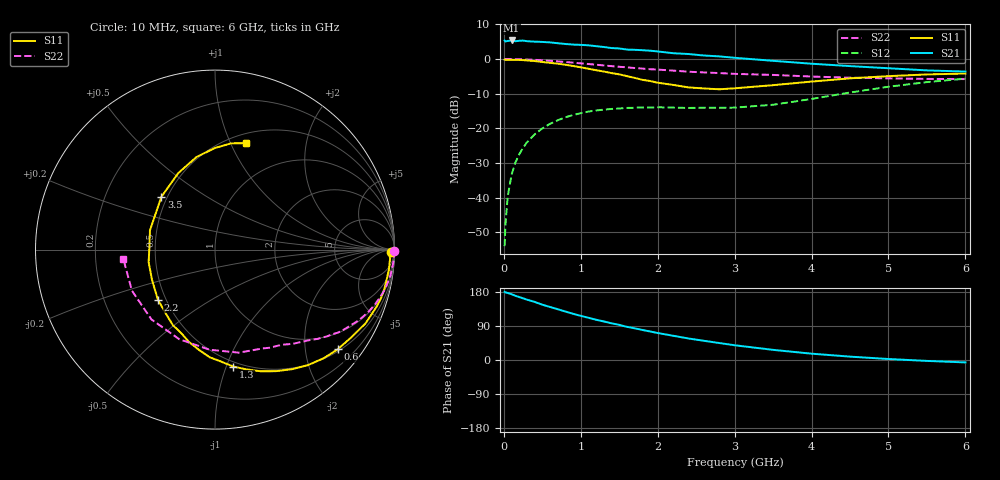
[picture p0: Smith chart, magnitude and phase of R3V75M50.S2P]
! SIEMENS Small Signal Semiconductors
! BFR181
! Si NPN RF Bipolar Junction Transistor in SOT23
! VCE = 0.75 V  IC = 0.5 mA
! Common Emitter S-Parameters:  May  1996
# GHz  S  MA  R  50
!  f  S11  S21  S12  S22
! GHz  MAG  ANG  MAG  ANG  MAG  ANG  MAG  ANG
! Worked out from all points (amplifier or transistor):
!   36 points, 10 MHz to 6 GHz, reference 50 ohm
!   highest |S21| = 5.3 dB at 100 MHz (marker M1)
!   |S21| within 3 dB of that: start of sweep to 1.923 GHz
!   unconditionally stable (mu >= 1): 2.261 GHz to 4.407 GHz
!   at 250 MHz: K = 0.12, MSG = 15.5 dB, |S12| = -25.6 dB
!   at 1.4 GHz: K = 0.65, MSG = 8.8 dB, |S12| = -14.4 dB
!   at 6 GHz: K = 0.98, MSG = 1.0 dB, |S12| = -5.7 dB
!   S11 on the Smith chart (normalised r, x): 10 MHz: 75, -48; 600 MHz: 0.55, -2.72; 1.3 GHz: 0.46, -1.06; 2.2 GHz: 0.45, -0.31; 3.5 GHz: 0.46, +0.33; 6 GHz: 0.60, +1.14
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0.01  0.9812 -0.7  1.847 179.8  0.002 91.0  0.999 -0.4
0.02  0.9718 -1.2  1.791 178.6  0.0039 87.7  0.994 -0.7
0.05  0.9767 -3.0  1.821 176.9  0.0104 86.7  0.9987 -1.6
0.1  0.9754 -6.5  1.851 173.7  0.0213 84.8  0.9974 -3.2
0.15  0.971 -9.7  1.805 169.4  0.0321 83.1  0.994 -5.1
0.2  0.969 -13.0  1.832 166.2  0.0423 80.8  0.9911 -6.5
0.3  0.9541 -19.7  1.807 159.3  0.0628 76.4  0.983 -9.9
0.5  0.9044 -32.5  1.762 145.9  0.0996 67.5  0.9573 -16.1
0.6  0.8808 -39.1  1.736 140.0  0.1162 63.1  0.9413 -19.1
0.9  0.7938 -57.0  1.615 121.9  0.1559 51.9  0.8867 -26.8
1.1  0.7235 -69.5  1.575 111.4  0.1745 45.6  0.8467 -31.6
1.3  0.6591 -81.2  1.49 101.7  0.1862 40.1  0.8069 -35.7
1.6  0.5658 -99.1  1.367 87.5  0.1971 33.8  0.7591 -40.9
1.8  0.5009 -112.3  1.34 79.3  0.2006 31.3  0.728 -43.9
2.2  0.423 -138.8  1.212 64.0  0.1994 27.9  0.6806 -50.5
2.4  0.3896 -154.2  1.18 56.8  0.197 28.3  0.6561 -53.7
2.8  0.3657 176.4  1.091 44.8  0.198 30.4  0.6271 -60.6
3.5  0.4194 135.4  0.941 26.8  0.2191 38.2  0.5893 -77.0
4  0.4726 115.7  0.855 16.7  0.2652 42.9  0.5588 -93.0
4.5  0.5262 101.3  0.79 8.9  0.3288 42.2  0.5375 -111.9
5.5  0.5991 81.3  0.685 -2.4  0.4644 30.7  0.5163 -153.7
6  0.6172 73.8  0.659 -6.4  0.5208 22.5  0.5133 -174.2
